| IBIS file stm32n657_vfbga142.ibs
[IBIS ver] 4.2
[File name] stm32n657_vfbga142.ibs
[File Rev] 1.1
[Date] 20-09-2024
[Source] Data Created at STMicroelectronics
[Notes]  File originated from ELDO simulations.
[Disclaimer]  This information is for modeling purpose only and is
   not guaranteed. The information is subject to change without
   notice.
[Copyright] Copyright 2024 STMicroelectronics Inc.
|   Component stm32n657_vfbga142
[Component] stm32n657_vfbga142
[Manufacturer] STMicroelectronics
[Package]
| variable   typ   min   max
R_pkg  0  NA  NA
L_pkg  0  NA  NA
C_pkg  0  NA  NA
[Pin]   signal_name   model_name
A1  PDR_ON  nc
A2  OTG2_ID  nc
A3  OTG2_HSDM  USB2_HS_IBIS
A4  NC  nc
A5  OTG1_HSDM  USB2_HS_IBIS
A6  OTG1_TXRTUNE  nc
A7  PH0-OSC_IN  isudq_tt
A8  PC8  io8_tt_i3c
A9  PC10  io8_tt_i3c
A10  PC12  io8_tt
A11  PE13  io8_tt_i3c
A12  PE7  io8_tt
A13  PE9  io8_tt
A14  PE0  io8_tt
A15  VSS  gnd
B1  PC15-OSC32_OUT  io8_tt_sw
B2  BOOT0  isudq_tt
B3  OTG2_HSDP  USB2_HS_IBIS
B4  OTG1_ID  nc
B5  OTG1_HSDP  USB2_HS_IBIS
B6  VDD33USB  power
B7  PH1-OSC_OUT  isudq_tt
B8  PC9  io8_tt_i3c
B9  PC11  io8_tt_i3c
B10  PH2  io8_tt
B11  PE12  io8_tt
B12  PD1  io8_tt
B13  PE10  io8_tt
B14  PE1  io8_tt
B15  PE2  io8_tt
C1  PC14-OSC32_IN  io8_tt_sw
C2  NRST  ioreset_tt_v18_1v8
C3  NC  nc
C13  PD8  io8_tt
C14  PB0  io8_tt
C15  PE3  io8_tt
D1  VBAT  power
D2  PWR_ON  io8_tt
D4  VDDA18USB  power
D5  OTG2_TXRTUNE  nc
D6  UCPD1_CC1  nc
D7  UCPD1_CC2  nc
D8  VDDIO4  power
D9  VSS  gnd
D10  PE14  io8_tt_i3c
D11  PE15  io8_tt_i3c
D12  PE8  io8_tt
D14  PN1  io8_tt
D15  PB6  io8_tt
E1  V08CAP  nc
E2  PC13  io8_tt_tamp
E4  VDDA18AON  nc
E12  PB7  io8_tt
E14  PN4  io8_tt
E15  PN8  io8_tt
F1  VDDA18PMU  nc
F2  VSSAPMU  nc
F3  VFBSMPS  nc
F4  VSSAON  nc
F12  VDD  power
F14  PN7  io8_tt
F15  PN5  io8_tt
G1  VSSSMPS  nc
G2  VSSSMPS  nc
G3  VSSSMPS  nc
G12  VDD  power
G14  PN9  io8_tt
G15  PN6  io8_tt
H1  VLXSMPS  nc
H2  VLXSMPS  nc
H3  VLXSMPS  nc
H12  VDD  power
H14  PN10  io8_tt
H15  PN2  io8_tt
J1  VDDSMPS  nc
J2  VDDSMPS  nc
J3  VDDSMPS  nc
J12  VSS  gnd
J14  PN11  io8_tt
J15  PN0  io8_tt
K1  PF4  io8_tt
K2  PF10  io8_tt
K3  PF5  io8_tt
K4  VDDA18PLL  nc
K12  VDDIO3  power
K14  PN12  io8_tt
K15  PN3  io8_tt
L1  PF2  io8_tt
L2  PF14  io8_tt
L4  PF3  io8_tt
L12  VDDIO3  power
L14  PB4  io8_tt
L15  PA15  io8_tt
M1  PF15  io8_tt
M2  PF7  io8_tt
M4  VSS  gnd
M5  VDDCORE  nc
M6  VDDCORE  nc
M7  VDDCORE  nc
M8  VDDCORE  nc
M9  VDDCORE  nc
M10  VSS  gnd
M11  PA8  io8_tt_i3c
M12  VSS  gnd
M14  PG2  io8_tt
M15  PB5  io8_tt_i3c
N1  PF8  io8_tt
N2  PF11  io8_tt
N3  PF13  io8_tt
N13  PB12  io8_tt_i3c
N14  PB11  io8_tt_i3c
N15  PB10  io8_tt_i3c
P1  PF12  io8_tt
P2  VREFP  nc
P3  VSSA  nc
P4  CSI_D1N  DPHY_IBIS_L1
P5  CSI_CKN  DPHY_IBIS_L1
P6  CSI_D0N  DPHY_IBIS_L1
P7  CSI_REXT  nc
P8  VDDCSI  nc
P9  PG14  io8_tt
P10  PA12  io8_tt
P11  PA9  io8_tt_i3c
P12  PA2  io8_tt
P13  PA6  io8_tt_i3c
P14  PA1  io8_tt
P15  PG10  io8_tt
R1  VSS  gnd
R2  VREFM  nc
R3  VDDA18ADC  nc
R4  CSI_D1P  DPHY_IBIS_L1
R5  CSI_CKP  DPHY_IBIS_L1
R6  CSI_D0P  DPHY_IBIS_L1
R7  VDDA18CSI  power
R8  PA14  io8_tt
R9  PA13  io8_tt
R10  PA11  io8_tt
R11  PA10  io8_tt
R12  PA5  io8_tt_i3c
R13  PG13  io8_tt
R14  PA0  io8_tt
R15  VSS  gnd
[Package Model]   486-fcvfbga-8x8-142-240308
[Pin Mapping]   pulldown_ref   pullup_ref   | Comment
A1  nc  nc
A2  nc  nc
A3  gnd  VDD33USB
A4  nc  nc
A5  gnd  VDD33USB
A6  nc  nc
A7  gnd  VDD
A8  gnd  VDDIO4
A9  gnd  VDDIO4
A10  gnd  VDDIO4
A11  gnd  VDD
A12  gnd  VDD
A13  gnd  VDD
A14  gnd  VDD
A15  gnd  nc
B1  gnd  VSW
B2  gnd  VDD
B3  gnd  VDD33USB
B4  nc  nc
B5  gnd  VDD33USB
B6  nc  VDD33USB
B7  gnd  VDD
B8  gnd  VDDIO4
B9  gnd  VDDIO4
B10  gnd  VDDIO4
B11  gnd  VDD
B12  gnd  VDD
B13  gnd  VDD
B14  gnd  VDD
B15  gnd  VDD
C1  gnd  VSW
C2  gnd  VDD
C3  nc  nc
C13  gnd  VDD
C14  gnd  VDD
C15  gnd  VDD
D1  nc  VSW
D2  gnd  VDD
D4  nc  VDDA18USB
D5  nc  nc
D6  nc  nc
D7  nc  nc
D8  nc  VDDIO4
D9  gnd  nc
D10  gnd  VDD
D11  gnd  VDD
D12  gnd  VDD
D14  gnd  VDDIO3
D15  gnd  VDD
E1  nc  nc
E2  gnd  VSW
E4  nc  nc
E12  gnd  VDD
E14  gnd  VDDIO3
E15  gnd  VDDIO3
F1  nc  nc
F2  nc  nc
F3  nc  nc
F4  nc  nc
F12  nc  VDD
F14  gnd  VDDIO3
F15  gnd  VDDIO3
G1  nc  nc
G2  nc  nc
G3  nc  nc
G12  nc  VDD
G14  gnd  VDDIO3
G15  gnd  VDDIO3
H1  nc  nc
H2  nc  nc
H3  nc  nc
H12  nc  VDD
H14  gnd  VDDIO3
H15  gnd  VDDIO3
J1  nc  nc
J2  nc  nc
J3  nc  nc
J12  gnd  nc
J14  gnd  VDDIO3
J15  gnd  VDDIO3
K1  gnd  VDD
K2  gnd  VDD
K3  gnd  VDD
K4  nc  nc
K12  nc  VDDIO3
K14  gnd  VDDIO3
K15  gnd  VDDIO3
L1  gnd  VDD
L2  gnd  VDD
L4  gnd  VDD
L12  nc  VDDIO3
L14  gnd  VDD
L15  gnd  VDD
M1  gnd  VDD
M2  gnd  VDD
M4  gnd  nc
M5  nc  nc
M6  nc  nc
M7  nc  nc
M8  nc  nc
M9  nc  nc
M10  gnd  nc
M11  gnd  VDD
M12  gnd  nc
M14  gnd  VDD
M15  gnd  VDD
N1  gnd  VDD
N2  gnd  VDD
N3  gnd  VDD
N13  gnd  VDD
N14  gnd  VDD
N15  gnd  VDD
P1  gnd  VDD
P2  nc  nc
P3  nc  nc
P4  gnd  VDDA18CSI
P5  gnd  VDDA18CSI
P6  gnd  VDDA18CSI
P7  nc  nc
P8  nc  nc
P9  gnd  VDD
P10  gnd  VDD
P11  gnd  VDD
P12  gnd  VDD
P13  gnd  VDD
P14  gnd  VDD
P15  gnd  VDD
R1  gnd  nc
R2  nc  nc
R3  nc  nc
R4  gnd  VDDA18CSI
R5  gnd  VDDA18CSI
R6  gnd  VDDA18CSI
R7  nc  VDDA18CSI
R8  gnd  VDD
R9  gnd  VDD
R10  gnd  VDD
R11  gnd  VDD
R12  gnd  VDD
R13  gnd  VDD
R14  gnd  VDD
R15  gnd  nc
[Diff Pin]  inv_pin  vdiff  tdelay_typ  tdelay_min  tdelay_max
R5  P5  NA  NA  NA  NA
R6  P6  NA  NA  NA  NA
R4  P4  NA  NA  NA  NA
B5  A5  NA  NA  NA  NA
B3  A3  NA  NA  NA  NA
[Model Selector] DPHY_IBIS_L1
DPHY_RX_2P5G_L1   DPHY HSRX model at 2.5Gbps for lane 1
DPHY_RX_1P5G_L1   DPHY HSRX model at 1.5Gbps for lane 1
[Model Selector] io8_tt
io8_tt_ls_3v3 "GPIO - 3V tolerant - low speed - 3.3V range"
io8_tt_ms_3v3 "GPIO - 3V tolerant - med speed - 3.3V range"
io8_tt_fs_3v3 "GPIO - 3V tolerant - fast speed - 3.3V range"
io8_tt_hs_3v3 "GPIO - 3V tolerant - high speed - 3.3V range"
io8_tt_hslv_ls_1v8 "GPIO low voltage optimization - 3V tolerant - low speed - 1.8V range"
io8_tt_hslv_ms_1v8 "GPIO low voltage optimization - 3V tolerant - med speed - 1.8V range"
io8_tt_hslv_fs_1v8 "GPIO low voltage optimization - 3V tolerant - fast speed - 1.8V range"
io8_tt_hslv_hs_1v8 "GPIO low voltage optimization - 3V tolerant - high speed - 1.8V range"
[Model Selector] io8_tt_i3c
io8_tt_ls_3v3 "GPIO - 3V tolerant - low speed - 3.3V range"
io8_tt_ms_3v3 "GPIO - 3V tolerant - med speed - 3.3V range"
io8_tt_fs_3v3 "GPIO - 3V tolerant - fast speed - 3.3V range"
io8_tt_hs_3v3 "GPIO - 3V tolerant - high speed - 3.3V range"
io8_tt_hslv_ls_1v8 "GPIO low voltage optimization - 3V tolerant - low speed - 1.8V range"
io8_tt_hslv_ms_1v8 "GPIO low voltage optimization - 3V tolerant - med speed - 1.8V range"
io8_tt_hslv_fs_1v8 "GPIO low voltage optimization - 3V tolerant - fast speed - 1.8V range"
io8_tt_hslv_hs_1v8 "GPIO low voltage optimization - 3V tolerant - high speed - 1.8V range"
io8_tt_i3c_ls_3v3 "GPIO with I3C open-drain - 3V tolerant - low speed - 3.3V range"
io8_tt_i3c_ms_3v3 "GPIO with I3C open-drain - 3V tolerant - med speed - 3.3V range"
io8_tt_i3c_fs_3v3 "GPIO with I3C open-drain - 3V tolerant - fast speed - 3.3V range"
io8_tt_i3c_hs_3v3 "GPIO with I3C open-drain - 3V tolerant - high speed - 3.3V range"
io8_tt_hslv_i3c_ls_1v8 "GPIO low voltage optimization with I3C open-drain - 3V tolerant - low speed - 1.8V range"
io8_tt_hslv_i3c_ms_1v8 "GPIO low voltage optimization with I3C open-drain - 3V tolerant - med speed - 1.8V range"
io8_tt_hslv_i3c_fs_1v8 "GPIO low voltage optimization with I3C open-drain - 3V tolerant - fast speed - 1.8V range"
io8_tt_hslv_i3c_hs_1v8 "GPIO low voltage optimization with I3C open-drain - 3V tolerant - high speed - 1.8V range"
io8_tt_i3c_fmp_3v3 "GPIO with I3C fm+ open-drain - 3V tolerant - 3.3V range"
[Model Selector] io8_tt_sw
io8_tt_sw_3v3 "Input Buffer - 3V tolerant - 3.3V range"
io8_tt_sw_1v8 "Input Buffer - 3V tolerant - 1.8V range"
[Model Selector] io8_tt_tamp
io8_tt_ls_3v3 "GPIO - 3V tolerant - low speed - 3.3V range"
io8_tt_ms_3v3 "GPIO - 3V tolerant - med speed - 3.3V range"
io8_tt_fs_3v3 "GPIO - 3V tolerant - fast speed - 3.3V range"
io8_tt_hs_3v3 "GPIO - 3V tolerant - high speed - 3.3V range"
io8_tt_hslv_ls_1v8 "GPIO low voltage optimization - 3V tolerant - low speed - 1.8V range"
io8_tt_hslv_ms_1v8 "GPIO low voltage optimization - 3V tolerant - med speed - 1.8V range"
io8_tt_hslv_fs_1v8 "GPIO low voltage optimization - 3V tolerant - fast speed - 1.8V range"
io8_tt_hslv_hs_1v8 "GPIO low voltage optimization - 3V tolerant - high speed - 1.8V range"
io8_tt_tamp_3v3 "IO tamper - 3V tolerant - 3.3V range"
io8_tt_tamp_1v8 "IO tamper - 3V tolerant - 1.8V range"
|[Model Selector] ioreset_tt_v18
|ioreset_tt_v18_1v8 "Reset PAD - 3V tolerant - 1.8V range"
[Model Selector] isudq_tt
isudq_tt_3v3 "Input Buffer - 3V tolerant - 3.3V range"
isudq_tt_1v8 "Input Buffer - 3V tolerant - 1.8V range"
[Model Selector] USB2_HS_IBIS
USB2_HSRX   USB2 HSRX model
USB2_HSTX_00_0_01_0011_11   TuningBits_AMP_PULSE_RISE_REF_XV=00_0_01_0011_11
USB2_HSTX_00_0_10_0101_11   TuningBits_AMP_PULSE_RISE_REF_XV=00_0_10_0101_11
USB2_HSTX_00_0_11_0111_11   TuningBits_AMP_PULSE_RISE_REF_XV=00_0_11_0111_11
USB2_HSTX_00_1_01_0011_11   TuningBits_AMP_PULSE_RISE_REF_XV=00_1_01_0011_11
USB2_HSTX_00_1_10_0101_11   TuningBits_AMP_PULSE_RISE_REF_XV=00_1_10_0101_11
USB2_HSTX_00_1_11_0111_11   TuningBits_AMP_PULSE_RISE_REF_XV=00_1_11_0111_11
USB2_HSTX_01_0_01_0011_11   TuningBits_AMP_PULSE_RISE_REF_XV=01_0_01_0011_11
USB2_HSTX_01_0_10_0101_11   TuningBits_AMP_PULSE_RISE_REF_XV=01_0_10_0101_11
USB2_HSTX_01_0_11_0111_11   TuningBits_AMP_PULSE_RISE_REF_XV=01_0_11_0111_11
USB2_HSTX_01_1_01_0011_11   TuningBits_AMP_PULSE_RISE_REF_XV=01_1_01_0011_11
USB2_HSTX_01_1_10_0101_11   TuningBits_AMP_PULSE_RISE_REF_XV=01_1_10_0101_11
USB2_HSTX_01_1_11_0111_11   TuningBits_AMP_PULSE_RISE_REF_XV=01_1_11_0111_11
USB2_HSTX_10_0_01_0011_11   TuningBits_AMP_PULSE_RISE_REF_XV=10_0_01_0011_11
USB2_HSTX_10_0_10_0101_11   TuningBits_AMP_PULSE_RISE_REF_XV=10_0_10_0101_11
USB2_HSTX_10_0_11_0111_11   TuningBits_AMP_PULSE_RISE_REF_XV=10_0_11_0111_11
USB2_HSTX_10_1_01_0011_11   TuningBits_AMP_PULSE_RISE_REF_XV=10_1_01_0011_11
USB2_HSTX_10_1_10_0101_11   TuningBits_AMP_PULSE_RISE_REF_XV=10_1_10_0101_11
USB2_HSTX_10_1_11_0111_11   TuningBits_AMP_PULSE_RISE_REF_XV=10_1_11_0111_11
[Define Package Model]  486-fcvfbga-8x8-142-240308
[Manufacturer]  unknown
[OEM]  unknown
[Description]  unknown
[Number Of Pins]  122
[Pin Numbers]
| Pin Name Terminal   Net Name   Starting Node   Ending Node
B2 | BOOT0
P5 | CSI_CKN
R5 | CSI_CKP
P6 | CSI_D0N
R6 | CSI_D0P
P4 | CSI_D1N
R4 | CSI_D1P
P7 | CSI_REXT
C2 | NRST
A5 | OTG1_HSDM
B5 | OTG1_HSDP
B4 | OTG1_ID
A6 | OTG1_TXRTUNE
A4 | NC
A3 | OTG2_HSDM
B3 | OTG2_HSDP
A2 | OTG2_ID
D5 | OTG2_TXRTUNE
C3 | NC
R14 | PA0
P14 | PA1
P12 | PA2
R12 | PA5
P13 | PA6
M11 | PA8
P11 | PA9
R11 | PA10
R10 | PA11
P10 | PA12
R9 | PA13
R8 | PA14
L15 | PA15
C14 | PB0
L14 | PB4
M15 | PB5
D15 | PB6
E12 | PB7
N15 | PB10
N14 | PB11
N13 | PB12
A8 | PC8
B8 | PC9
A9 | PC10
B9 | PC11
A10 | PC12
E2 | PC13
C1 | PC14-OSC32_IN
B1 | PC15-OSC32_OUT
B12 | PD1
C13 | PD8
A1 | PDR_ON
A14 | PE0
B14 | PE1
B15 | PE2
C15 | PE3
A12 | PE7
D12 | PE8
A13 | PE9
B13 | PE10
B11 | PE12
A11 | PE13
D10 | PE14
D11 | PE15
L1 | PF2
L4 | PF3
K1 | PF4
K3 | PF5
M2 | PF7
N1 | PF8
K2 | PF10
N2 | PF11
P1 | PF12
N3 | PF13
L2 | PF14
M1 | PF15
M14 | PG2
P15 | PG10
R13 | PG13
P9 | PG14
A7 | PH0-OSC_IN
B7 | PH1-OSC_OUT
B10 | PH2
J15 | PN0
D14 | PN1
H15 | PN2
K15 | PN3
E14 | PN4
F15 | PN5
G15 | PN6
F14 | PN7
E15 | PN8
G14 | PN9
H14 | PN10
J14 | PN11
K14 | PN12
D2 | PWR_ON
D6 | UCPD1_CC1
D7 | UCPD1_CC2
E1 | V08CAP
D1 | VBAT
B6 | VDD33USB
F12 | VDD
R3 | VDDA18ADC
E4 | VDDA18AON
R7 | VDDA18CSI
K4 | VDDA18PLL
F1 | VDDA18PMU
D4 | VDDA18USB
M5 | VDDCORE
P8 | VDDCSI
K12 | VDDIO3
D8 | VDDIO4
J1 | VDDSMPS
F3 | VFBSMPS
H1 | VLXSMPS
R2 | VREFM
P2 | VREFP
A15 | VSS
P3 | VSSA
F4 | VSSAON
F2 | VSSAPMU
G1 | VSSSMPS
|[Merged Pins]  F12
|G12  |  VDD
|H12  |  VDD
|[Merged Pins]  M5
|M6  |  VDDCORE
|M7  |  VDDCORE
|M8  |  VDDCORE
|M9  |  VDDCORE
|[Merged Pins]  K12
|L12  |  VDDIO3
|[Merged Pins]  J1
|J2  |  VDDSMPS
|J3  |  VDDSMPS
|[Merged Pins]  H1
|H2  |  VLXSMPS
|H3  |  VLXSMPS
|[Merged Pins]  A15
|D9  |  VSS
|J12  |  VSS
|M4  |  VSS
|M10  |  VSS
|M12  |  VSS
|R1  |  VSS
|R15  |  VSS
|[Merged Pins]  G1
|G2  |  VSSSMPS
|G3  |  VSSSMPS
[Model Data]
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[End Model Data]
[End Package Model]
|End [Component]
| Models and submodels in the file (45): DPHY_RX_1P5G_L1 (Input), DPHY_RX_2P5G_L1 (Input), io8_tt_fs_3v3 (I/O), io8_tt_hs_3v3 (I/O), io8_tt_hslv_fs_1v8 (I/O), io8_tt_hslv_hs_1v8 (I/O), io8_tt_hslv_i3c_fs_1v8 (I/O_open_drain), io8_tt_hslv_i3c_hs_1v8 (I/O_open_drain), io8_tt_hslv_i3c_ls_1v8 (I/O_open_drain), io8_tt_hslv_i3c_ms_1v8 (I/O_open_drain), io8_tt_hslv_ls_1v8 (I/O), io8_tt_hslv_ms_1v8 (I/O), io8_tt_i3c_fmp_3v3 (I/O_open_drain), io8_tt_i3c_fs_3v3 (I/O_open_drain), io8_tt_i3c_hs_3v3 (I/O_open_drain), io8_tt_i3c_ls_3v3 (I/O_open_drain), io8_tt_i3c_ms_3v3 (I/O_open_drain), io8_tt_ls_3v3 (I/O), io8_tt_ms_3v3 (I/O), io8_tt_sw_1v8 (I/O), io8_tt_sw_3v3 (I/O), io8_tt_tamp_1v8 (I/O), io8_tt_tamp_3v3 (I/O), ioreset_tt_v18_1v8 (I/O_open_drain), isudq_tt_1v8 (Input), isudq_tt_3v3 (Input), USB2_HSRX (Input), USB2_HSTX_00_0_01_0011_11 (Output), USB2_HSTX_00_0_10_0101_11 (Output), USB2_HSTX_00_0_11_0111_11 (Output), USB2_HSTX_00_1_01_0011_11 (Output), USB2_HSTX_00_1_10_0101_11 (Output), USB2_HSTX_00_1_11_0111_11 (Output), USB2_HSTX_01_0_01_0011_11 (Output), USB2_HSTX_01_0_10_0101_11 (Output), USB2_HSTX_01_0_11_0111_11 (Output), USB2_HSTX_01_1_01_0011_11 (Output), USB2_HSTX_01_1_10_0101_11 (Output), USB2_HSTX_01_1_11_0111_11 (Output), USB2_HSTX_10_0_01_0011_11 (Output), USB2_HSTX_10_0_10_0101_11 (Output), USB2_HSTX_10_0_11_0111_11 (Output), USB2_HSTX_10_1_01_0011_11 (Output), USB2_HSTX_10_1_10_0101_11 (Output), USB2_HSTX_10_1_11_0111_11 (Output)
